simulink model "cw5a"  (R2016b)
settings: Solver=FixedStepAuto  StartTime=0.0  StopTime=100  FixedStep=0.01  RelTol=1e-3
libraries: simulink x1, fuzblock x1

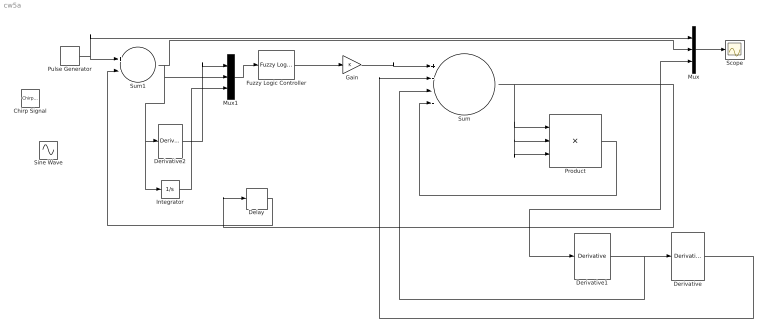
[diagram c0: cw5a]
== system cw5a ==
  Chirp Signal : simulink/Sources/Chirp Signal  f1=0.02  T=100  f2=0.2
  Delay : Delay  DelayLength=1  InitialCondition=0
  Derivative : Derivative
  Derivative1 : Derivative
  Derivative2 : Derivative
  Fuzzy Logic Controller : fuzblock/Fuzzy Logic  Controller  fis='pid2.fis'
  Gain : Gain
  Integrator : Integrator
  Mux : Mux  Inputs=3
  Mux1 : Mux  Inputs=3
  Product : Product  Inputs=3
  Pulse Generator : DiscretePulseGenerator  PulseType=Time based  Period=10  PulseWidth=50
  Scope : Scope
  Sine Wave : Sin  Frequency=0.11  SampleTime=0
  Sum : Sum  Inputs=+---
  Sum1 : Sum  Inputs=+-
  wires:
  Mux/1 -> Scope/1
  Product/1 -> Sum/4
  Sum/1 -> Product/3, Product/2, Product/1, Mux/3, Derivative1/1, Delay/1
  Derivative1/1 -> Sum/3, Derivative/1
  Derivative/1 -> Sum/2
  Pulse Generator/1 -> Mux/1, Sum1/1
  Sum1/1 -> Mux1/2, Integrator/1, Derivative2/1, Mux/2
  Delay/1 -> Sum1/2
  Mux1/1 -> Fuzzy Logic Controller/1
  Gain/1 -> Sum/1
  Fuzzy Logic Controller/1 -> Gain/1
  Derivative2/1 -> Mux1/1
  Integrator/1 -> Mux1/3
